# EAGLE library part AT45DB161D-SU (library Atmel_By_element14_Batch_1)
16-megabit DataFlash
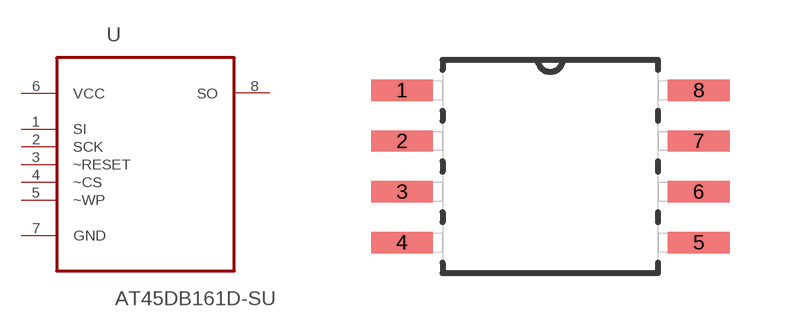
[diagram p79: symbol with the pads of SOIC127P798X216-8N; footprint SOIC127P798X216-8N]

Designator prefix U

## AT45DB161D-SU (MPN: AT45DB161D-SU; OC_FARNELL: 1455040; OC_NEWARK: 58M3838; PACKAGE: SOIC-8; SUPPLIER: Atmel)  [SOIC127P798X216-8N]
1  SI  in
2  SCK  in
3  ~RESET  in
4  ~CS  in
5  ~WP  in
6  VCC  pwr
7  GND  pas
8  SO  out

## Footprint SOIC127P798X216-8N (pad centres in mm)
smd 1.549 x 0.533: 1 -3.708,1.905; 2 -3.708,0.635; 3 -3.708,-0.635; 4 -3.708,-1.905; 5 3.708,-1.905; 6 3.708,-0.635; 7 3.708,0.635; 8 3.708,1.905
